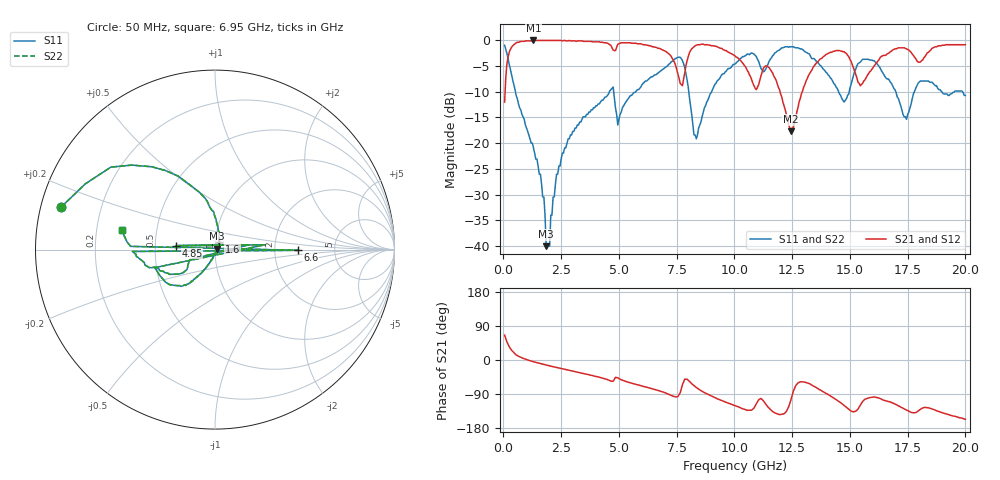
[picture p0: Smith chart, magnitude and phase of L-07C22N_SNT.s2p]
#	mhz	s	ma	r	50
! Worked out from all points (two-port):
!   400 points, 50 MHz to 20 GHz, reference 50 ohm
!   highest |S21| = -0.09 dB at 1.3 GHz (marker M1); lowest = -17.7 dB at 12.45 GHz (marker M2)
!   |S21| within 3 dB of the highest: 213.6 MHz to 7.248 GHz (7.034 GHz wide, 189 % of centre); 8.009 GHz to 10.02 GHz (2.013 GHz wide, 22.3 % of centre)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
!   lowest |S11| = -40.0 dB at 1.85 GHz (marker M3), VSWR 1.02, Z = 50.9 + j0.465 ohm
!   |S11| at or under -10 dB: 516.5 MHz to 4.591 GHz (4.074 GHz wide, 160 % of centre); 4.773 GHz to 5.731 GHz (958.6 MHz wide, 18.3 % of centre); 8.023 GHz to 9.016 GHz (993.2 MHz wide, 11.7 % of centre)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
!   |S22| runs from -40.0 to -1.0 dB; largest |S21 - S12| = 0
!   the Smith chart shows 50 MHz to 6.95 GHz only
!   S11 on the Smith chart (normalised r, x): 50 MHz: 0.06, +0.13; 1.6 GHz: 1.04, +0.09; 4.85 GHz: 0.64, +0.03; 6.6 GHz: 2.70, -0.03; 6.95 GHz: 0.31, +0.09
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50  0.89 164.6  0.25 65.7  0.25 65.7  0.89 164.6
450  0.37 109.6  0.9 19.9  0.9 19.9  0.37 109.6
1300  0.09 74.8  0.99 -4.5  0.99 -4.5  0.09 74.8
1600  0.05 62.5  0.99 -9.5  0.99 -9.5  0.05 62.5
1850  0.01 27.2  0.99 -13.3  0.99 -13.3  0.01 27.2
3400  0.17 -122.2  0.98 -34.9  0.98 -34.9  0.17 -122.2
4750  0.35 -163.3  0.8 -56.1  0.8 -56.1  0.35 -163.3
4800  0.28 5.5  0.79 -51.0  0.79 -51.0  0.28 5.5
4850  0.22 174.3  0.79 -45.8  0.79 -45.8  0.22 174.3
6550  0.46 -178.7  0.85 -77.8  0.85 -77.8  0.46 -178.7
6600  0.46 -0.5  0.85 -78.7  0.85 -78.7  0.46 -0.5
6650  0.47 177.8  0.84 -79.6  0.84 -79.6  0.47 177.8
6700  0.48 176.5  0.83 -80.4  0.83 -80.4  0.48 176.5
6950  0.53 168.3  0.79 -85.3  0.79 -85.3  0.53 168.3
7700  0.66 110.2  0.37 -76.0  0.37 -76.0  0.66 110.2
8350  0.11 121.6  0.89 -72.6  0.89 -72.6  0.11 121.6
10050  0.59 137.4  0.69 -121.0  0.69 -121.0  0.59 137.4
12450  0.86 62.5  0.13 -104.4  0.13 -104.4  0.86 62.5
13350  0.66 27.3  0.51 -66.3  0.51 -66.3  0.66 27.3
14950  0.3 31.2  0.69 -129.8  0.69 -129.8  0.3 31.2
16700  0.41 -27.2  0.75 -110.1  0.75 -110.1  0.41 -27.2
20000  0.29 -83.1  0.9 -156.4  0.9 -156.4  0.29 -83.1
